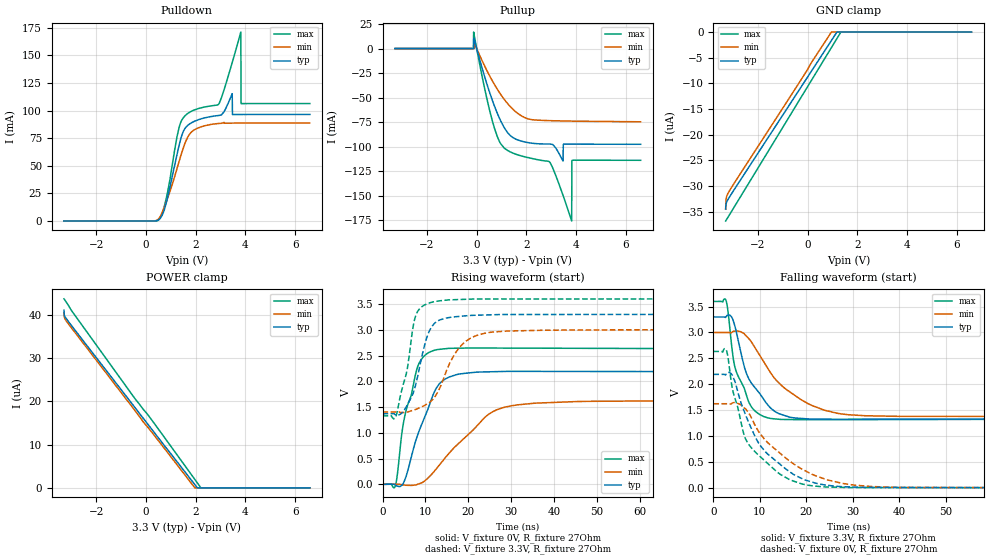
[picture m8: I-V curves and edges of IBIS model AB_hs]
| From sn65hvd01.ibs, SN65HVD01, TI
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|   Model
[Model]   AB_hs
Model_type   I/O
Polarity   Non-Inverting
Enable   Active-Low
Vinl = 0.99
Vinh = 2.31
Vmeas = 1.65
Vref = 1.65
Cref = 1pF
Rref = 27
|   typ   min   max
C_comp   2.359pF   1.818pF   2.464pF
[Voltage Range]   3.3   3   3.6
[Temperature Range]   27   125   -40
[Pullup Reference]   3.3   3   3.6
[Pulldown Reference]   -0   -0   -0
[Power Clamp Reference]   3.3   3   3.6
[GND Clamp Reference]   -0   -0   -0
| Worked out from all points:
|   slope of the pulldown table from 0 to 0.495 V, typ, clamps not added: 608 ohm
|   slope of the pullup table from 0 to 0.495 V, typ, clamps not added: 11.6 ohm
|   falling waveform, V_fixture 3.3V, R_fixture 27Ohm: 20-80 % time 5.52ns typ, 9.71ns min, 3.67ns max; typ from 3.3 V to 1.33 V
|   rising waveform, V_fixture 0V, R_fixture 27Ohm: 20-80 % time 5.43ns typ, 11ns min, 3.71ns max; typ from 0 V to 2.19 V
|   rising waveform, V_fixture 3.3V, R_fixture 27Ohm: 20-80 % time 3.55ns typ, 5.82ns min, 2.99ns max; typ from 1.37 V to 3.3 V
|   falling waveform, V_fixture 0V, R_fixture 27Ohm: 20-80 % time 9ns typ, 11.4ns min, 7.24ns max; typ from 2.19 V to 0.001 V
[Pulldown]
|   Voltage   I(typ)   I(min)   I(max)
-3.29V    971.4nA    1.42uA     915.1nA
541.2mV   1.571mA    2.781mA    1.547mA
858mV     19.8mA     19.6mA     24.42mA
1.333V    68.19mA    53.72mA    84.45mA
1.601V    84.7mA     71.9mA     95.88mA
1.937V    90.18mA    82.44mA    100.5mA
2.937V    95.63mA    88.35mA    106.2mA
3.472V    115.3mA    88.68mA    143.5mA
3.482V    96.46mA    88.68mA    144.3mA
3.818V    96.51mA    88.71mA    171.2mA
3.828V    96.51mA    88.71mA    106.4mA
6.59V     96.53mA    88.76mA    106.4mA
[GND Clamp]
|   Voltage   I(typ)   I(min)   I(max)
-3.29V    -34.51uA   -34.54uA   -36.84uA
-3.28V    -33.74uA   -32.98uA   -36.76uA
-3.26V    -33.29uA   -32.24uA   -36.6uA
-3.221V   -32.85uA   -31.68uA   -36.29uA
-3.142V   -32.2uA    -30.98uA   -35.66uA
-132mV    -9.777uA   -8.336uA   -11.72uA
204.6mV   -7.277uA   -5.602uA   -9.046uA
957mV     -1.682uA   -32.01nA   -3.062uA
1.185V    0A         0A         -1.251uA
1.343V    0A         0A         0A
6.59V     0A         0A         0A
[Pullup]
|   Voltage   I(typ)   I(min)   I(max)
-3.29V    -1.81uA    -1.869uA   846.3nA
-132mV    615.2nA    897.1nA    864.2nA
-122.1mV  619.1nA    904.2nA    16.85mA
-112.2mV  10.8mA     910.4nA    15.47mA
927.3mV   -71.71mA   -45.34mA   -95.33mA
1.521V    -91.73mA   -63.42mA   -107.3mA
2.937V    -97.38mA   -73.51mA   -115.9mA
3.472V    -114.7mA   -73.83mA   -149.8mA
3.491V    -97.46mA   -73.84mA   -151.2mA
3.818V    -97.49mA   -73.99mA   -175.9mA
3.828V    -97.49mA   -73.99mA   -114.2mA
6.59V     -97.64mA   -74.69mA   -114mA
[POWER Clamp]
|   Voltage   I(typ)   I(min)   I(max)
-3.29V    41.06uA    40.44uA    43.66uA
-3.28V    40.04uA    39.6uA     43.58uA
-3.27V    39.8uA     39.34uA    43.5uA
-3.132V   38.58uA    38.04uA    42.33uA
-2.924V   37.01uA    36.47uA    40.44uA
-537.9mV  19.3uA     18.61uA    21.41uA
-112.2mV  16.13uA    15.31uA    18.21uA
214.5mV   13.7uA     13.04uA    15.86uA
1.967V    756.8nA    16.25nA    1.965uA
2.066V    21.54nA    0A         1.178uA
2.214V    0A         0A         0A
6.59V     0A         0A         0A
[Ramp]
R_load = 27
|   typ   min   max
dV/dt_r   1.31081/5.41776e-09   0.971551/1.10314e-08   1.57638/3.70288e-09
dV/dt_f   1.18121/5.49901e-09   0.973025/9.69578e-09   1.36243/3.64603e-09
[Falling Waveform]
V_fixture = 3.3V
V_fixture_min = 3V
V_fixture_max = 3.6V
R_fixture = 27Ohm
C_fixture = 0F
|   Time   V(typ)   V(min)   V(max)
0s        3.3V       3V         3.6V
2.641ns   3.291V     3V         3.636V
3.104ns   3.335V     3V         3.435V
3.862ns   3.307V     2.997V     2.801V
4.662ns   3.112V     3.027V     2.321V
7.702ns   2.092V     2.873V     1.639V
11.71ns   1.603V     2.308V     1.352V
18.75ns   1.341V     1.709V     1.316V
27.83ns   1.324V     1.424V     1.318V
100ns     1.331V     1.378V     1.329V
[Rising Waveform]
V_fixture = 0V
V_fixture_min = 0V
V_fixture_max = 0V
R_fixture = 27Ohm
C_fixture = 0F
|   Time   V(typ)   V(min)   V(max)
0s        209uV      167.2uV    258.3uV
2.95ns    -10.89mV   2.201mV    -41.75mV
4.833ns   18.29mV    -10.74mV   1.166V
8.479ns   1.024V     9.639mV    2.342V
12.01ns   1.778V     248.2mV    2.6V
14.03ns   2.012V     453.8mV    2.627V
17.16ns   2.127V     748.4mV    2.642V
24.61ns   2.184V     1.352V     2.645V
30.3ns    2.193V     1.528V     2.644V
100ns     2.185V     1.619V     2.628V
[Rising Waveform]
V_fixture = 3.3V
V_fixture_min = 3V
V_fixture_max = 3.6V
R_fixture = 27Ohm
C_fixture = 0F
|   Time   V(typ)   V(min)   V(max)
0s        1.368V     1.403V     1.329V
3.104ns   1.35V      1.406V     1.315V
5.48ns    1.495V     1.4V       2.127V
7.702ns   1.921V     1.454V     3.264V
9.69ns    2.663V     1.526V     3.477V
11.11ns   3.007V     1.6V       3.526V
13.24ns   3.188V     1.851V     3.561V
17.99ns   3.26V      2.661V     3.588V
23.82ns   3.287V     2.932V     3.597V
100ns     3.3V       3V         3.6V
[Falling Waveform]
|Gnd
V_fixture = 0V
V_fixture_min = 0V
V_fixture_max = 0V
R_fixture = 27Ohm
C_fixture = 0F
|   Time   V(typ)   V(min)   V(max)
0s        2.191V     1.624V     2.634V
2.795ns   2.203V     1.625V     2.661V
4.137ns   2.16V      1.64V      1.895V
6.563ns   1.494V     1.552V     1.033V
7.453ns   1.293V     1.465V     859.2mV
11.08ns   706.8mV    930.1mV    520.1mV
18.98ns   182.5mV    365.6mV    76.87mV
24.61ns   49.29mV    151.8mV    17.12mV
34.01ns   8.06mV     25.69mV    5.857mV
100ns     563.8uV    578.4uV    577.9uV
